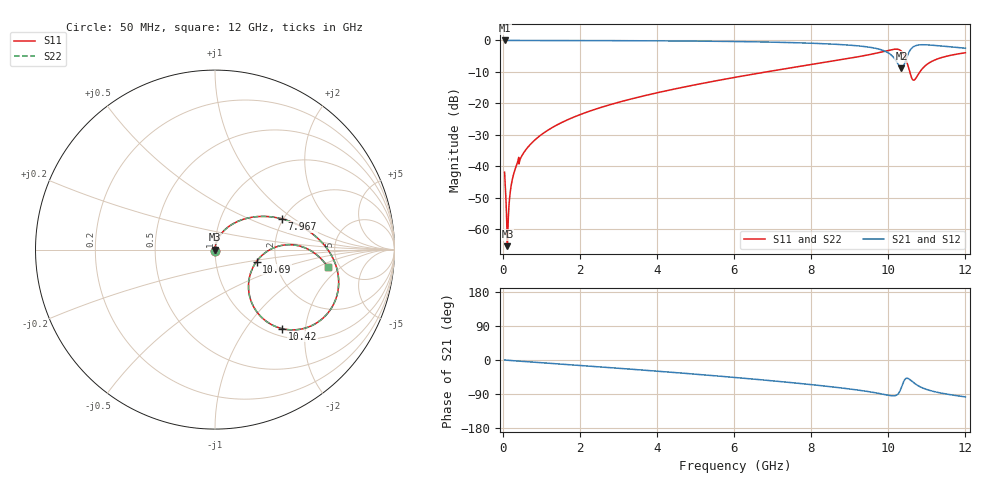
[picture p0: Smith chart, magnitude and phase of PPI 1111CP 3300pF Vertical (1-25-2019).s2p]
# GHz S MA R 50
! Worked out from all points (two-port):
!   1601 points, 50 MHz to 12 GHz, reference 50 ohm
!   highest |S21| = 0.00 dB at 50 MHz (marker M1); lowest = -8.8 dB at 10.34 GHz (marker M2)
!   |S21| within 3 dB of the highest: start of sweep to 9.828 GHz; 10.57 GHz to end of sweep
!   lowest |S11| = -65.4 dB at 124.7 MHz (marker M3), VSWR 1.00, Z = 50.1 + j0.0138 ohm
!   |S11| at or under -10 dB: start of sweep to 6.835 GHz; 10.56 GHz to 10.82 GHz (263.7 MHz wide, 2.47 % of centre)
!   |S22| runs from -65.4 to -2.8 dB; largest |S21 - S12| = 0
!   S11 on the Smith chart (normalised r, x): 50 MHz: 1.00, -0.02; 7.967 GHz: 1.97, +0.81; 10.42 GHz: 1.14, -1.51; 10.69 GHz: 1.58, -0.22; 12 GHz: 4.04, -1.34
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0.05  0.008042 -87.2  0.9996 0.2  0.9996 0.2  0.008042 -87.2
0.079875  0.003494 -83.1  0.9996 -0.2  0.9996 -0.2  0.003494 -83.1
0.1246875  0.0005379 14.9  0.9995 -0.7  0.9995 -0.7  0.0005379 14.9
0.1620312  0.002312 74.6  0.9994 -1.0  0.9994 -1.0  0.002312 74.6
0.2217813  0.005017 81.0  0.9993 -1.5  0.9993 -1.5  0.005017 81.0
0.3114062  0.008582 82.7  0.9992 -2.1  0.9992 -2.1  0.008582 82.7
0.6026875  0.01841 82.6  0.9988 -4.3  0.9988 -4.3  0.01841 82.6
1.162844  0.03716 79.6  0.9979 -8.3  0.9979 -8.3  0.03716 79.6
2.044156  0.06761 73.8  0.9958 -14.7  0.9958 -14.7  0.06761 73.8
4.038312  0.1489 59.3  0.986 -29.7  0.986 -29.7  0.1489 59.3
6.025  0.2593 43.1  0.9618 -46.1  0.9618 -46.1  0.2593 43.1
7.966875  0.4111 24.6  0.9052 -64.6  0.9052 -64.6  0.4111 24.6
8.019156  0.416 24.0  0.9029 -65.1  0.9029 -65.1  0.416 24.0
9.348594  0.5695 7.0  0.8045 -81.3  0.8045 -81.3  0.5695 7.0
10.01331  0.6979 -11.0  0.6271 -93.2  0.6271 -93.2  0.6979 -11.0
10.2075  0.7275 -24.3  0.4705 -93.0  0.4705 -93.0  0.7275 -24.3
10.34194  0.6753 -39.7  0.3612 -72.0  0.3612 -72.0  0.6753 -39.7
10.41662  0.5784 -49.6  0.4216 -53.4  0.4216 -53.4  0.5784 -49.6
10.54359  0.3358 -54.2  0.6642 -50.5  0.6642 -50.5  0.3358 -54.2
10.69297  0.2407 -16.0  0.8182 -62.4  0.8182 -62.4  0.2407 -16.0
11.13363  0.4665 2.6  0.8405 -81.9  0.8405 -81.9  0.4665 2.6
12  0.6373 -8.9  0.7531 -97.4  0.7531 -97.4  0.6373 -8.9
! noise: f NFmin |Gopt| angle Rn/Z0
0.05  0.0004128  0.8784  0.2698  0.0007345
1.372  0.00438  0.7142  7.135  0.003013
2.701  0.007305  0.6738  13.84  0.004255
4.031  0.01005  0.6558  20.34  0.005402
5.36  0.01291  0.6523  26.61  0.006704
6.682  0.01625  0.6631  32.67  0.008536
8.012  0.02152  0.6985  38.79  0.01247
9.341  0.04007  0.8058  45.57  0.03655
10.67  0.1373  0.9328  52.26  0.3669
12  0.0454  0.7977  56.52  0.03617
